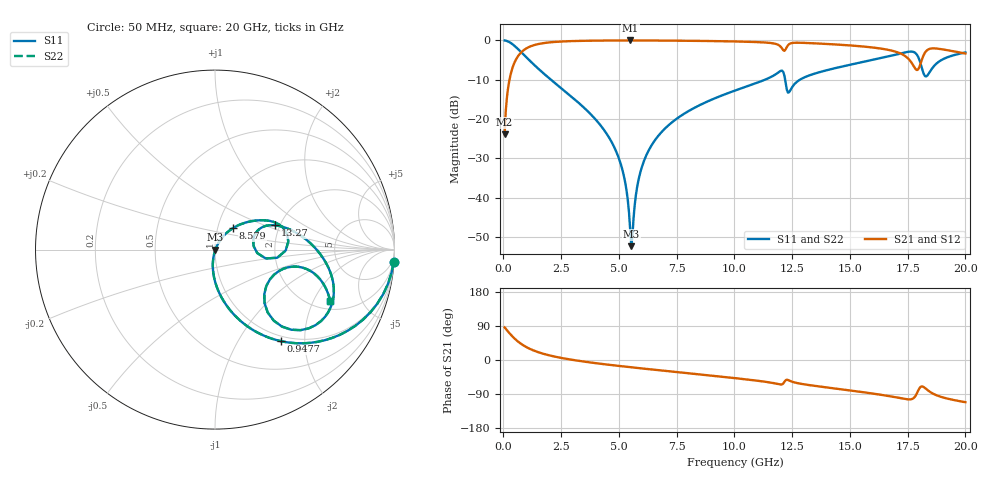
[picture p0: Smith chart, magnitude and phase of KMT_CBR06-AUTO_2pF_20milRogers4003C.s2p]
! Data measured by Modelithics Inc. support@modelithics.com 813-866-6335
! KEMET CBR06-AUTO 2pF, Pad Width= 0.851mm, Pad Length= 0.64mm, Pad Gap= 0.62mm, 20mil Rogers 4003C substrate Data, January 2022
# hz S ma R 50
! 2 Port Network Data from SP1.SP block
! freq  magS11  angS11  magS21  angS21  magS12  angS12  magS22  angS22
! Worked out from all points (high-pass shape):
!   401 points, 50 MHz to 20 GHz, reference 50 ohm
!   highest |S21| = -0.02 dB at 5.486 GHz (marker M1); lowest = -23.9 dB at 50 MHz (marker M2)
!   |S21| within 3 dB of the highest: 772.2 MHz to 17.06 GHz (16.29 GHz wide, 183 % of centre); 18.26 GHz to 19.71 GHz (1.451 GHz wide, 7.64 % of centre)
!   lowest |S11| = -52.4 dB at 5.536 GHz (marker M3), VSWR 1.00, Z = 50.2 - j0.118 ohm
!   |S11| at or under -10 dB: 2.055 GHz to 11.33 GHz (9.272 GHz wide, 139 % of centre); 12.2 GHz to 12.84 GHz (641.4 MHz wide, 5.12 % of centre)
!   |S22| runs from -52.4 to 0.0 dB; largest |S21 - S12| = 0
!   S11 on the Smith chart (normalised r, x): 50 MHz: 1, -30; 947.8 MHz: 0.92, -1.54; 8.579 GHz: 1.18, +0.29; 13.27 GHz: 1.89, +0.59; 20 GHz: 2.42, -2.72
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5e7  0.998 -3.8  0.06348 86.2  0.06348 86.2  0.998 -3.8
3.4925e8  0.913 -25.2  0.4071 64.7  0.4071 64.7  0.913 -25.2
9.4775e8  0.6275 -54.3  0.7773 35.5  0.7773 35.5  0.6275 -54.3
3.391625e9  0.1477 -92.6  0.9869 -3.4  0.9869 -3.4  0.1477 -92.6
4.887875e9  0.03816 -101.5  0.9968 -14.9  0.9968 -14.9  0.03816 -101.5
5.237e9  0.01751 -99.7  0.9973 -17.3  0.9973 -17.3  0.01751 -99.7
5.486375e9  0.00397 -72.4  0.9974 -18.9  0.9974 -18.9  0.00397 -72.4
5.53625e9  0.002406 -29.2  0.9974 -19.3  0.9974 -19.3  0.002406 -29.2
5.985125e9  0.02403 61.9  0.9971 -22.2  0.9971 -22.2  0.02403 61.9
6.73325e9  0.06252 60.6  0.9952 -27.0  0.9952 -27.0  0.06252 60.6
8.578625e9  0.1541 50.3  0.9847 -38.6  0.9847 -38.6  0.1541 50.3
1.0025e10  0.2299 41.2  0.9691 -47.9  0.9691 -47.9  0.2299 41.2
1.197012e10  0.4039 15.7  0.8483 -64.5  0.8483 -64.5  0.4039 15.7
1.22195e10  0.2871 -9.9  0.7712 -53.2  0.7712 -53.2  0.2871 -9.9
1.326688e10  0.3607 22.1  0.9229 -66.5  0.9229 -66.5  0.3607 22.1
1.336662e10  0.3692 21.3  0.9201 -67.3  0.9201 -67.3  0.3692 21.3
1.670825e10  0.629 -7.6  0.7526 -95.4  0.7526 -95.4  0.629 -7.6
1.7606e10  0.7204 -26.8  0.5512 -104.0  0.5512 -104.0  0.7204 -26.8
1.795512e10  0.6167 -46.4  0.4279 -80.8  0.4279 -80.8  0.6167 -46.4
1.82045e10  0.3701 -42.1  0.6608 -71.7  0.6608 -71.7  0.3701 -42.1
1.86035e10  0.4577 -11.9  0.7913 -88.9  0.7913 -88.9  0.4577 -11.9
2e10  0.702 -24.0  0.6803 -111.4  0.6803 -111.4  0.702 -24.0
